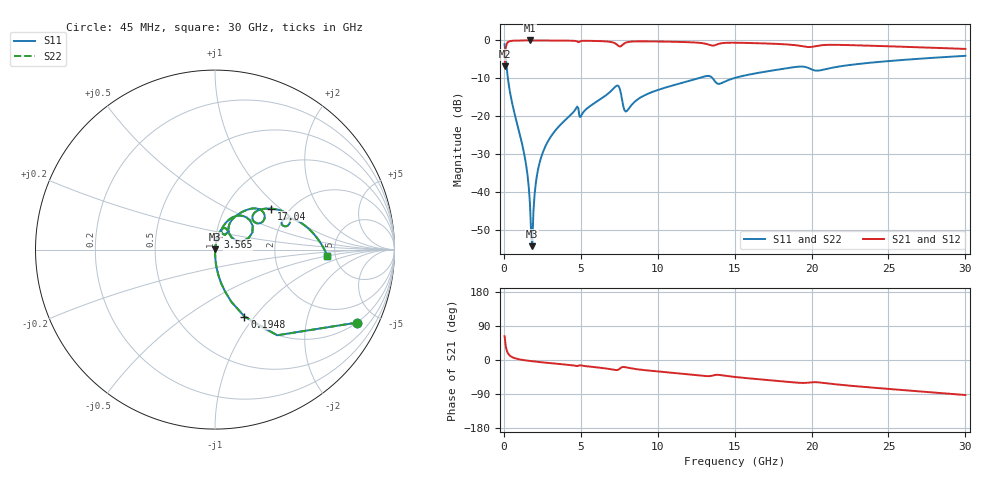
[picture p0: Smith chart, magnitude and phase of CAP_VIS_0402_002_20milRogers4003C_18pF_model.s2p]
! S-parameter model data by Modelithics Inc.  support@modelithics.com  813-866-6335  Tampa FL USA
! S-Parameter data specifications:
! Substrate: 20-mil Rogers 4003C, substrate thickness, H=0.508mm, Dielectric constant, Er=3.75
! PCB Mounting Pad Footprint: Pad width, PadW=0.50mm , Pad length, PadL=0.50mm , Pad gap, PadG (edge-to-edge)=0.40mm , Reference planes=1.4mm apart
! Created Wed Nov 18 12:52:21 2015
# hz S ma R 50
! 2 Port Network Data from SP1.SP block
! freq  magS11  angS11  magS21  angS21  magS12  angS12  magS22  angS22
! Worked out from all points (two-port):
!   401 points, 45 MHz to 30 GHz, reference 50 ohm
!   highest |S21| = -0.01 dB at 1.693 GHz (marker M1); lowest = -6.8 dB at 45 MHz (marker M2)
!   |S21| within 3 dB of the highest: 102.5 MHz to end of sweep
!   lowest |S11| = -54.3 dB at 1.842 GHz (marker M3), VSWR 1.00, Z = 50.1 + j0.128 ohm
!   |S11| at or under -10 dB: 259.5 MHz to 12.65 GHz (12.39 GHz wide, 192 % of centre); 13.56 GHz to 14.93 GHz (1.369 GHz wide, 9.61 % of centre)
!   |S22| runs from -54.3 to -1.0 dB; largest |S21 - S12| = 0
!   S11 on the Smith chart (normalised r, x): 45 MHz: 1.00, -3.90; 194.8 MHz: 1.00, -0.89; 3.565 GHz: 1.02, +0.15; 17.04 GHz: 1.63, +0.87; 30 GHz: 4.29, -0.47
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4.5e7  0.8901 -27.2  0.4556 62.8  0.4556 62.8  0.8901 -27.2
1.94775e8  0.4076 -66.2  0.9127 23.7  0.9127 23.7  0.4076 -66.2
4.194375e8  0.1947 -79.3  0.9802 10.5  0.9802 10.5  0.1947 -79.3
1.392975e9  0.02614 -88.3  0.9984 -0.9  0.9984 -0.9  0.02614 -88.3
1.54275e9  0.01602 -87.3  0.9986 -1.8  0.9986 -1.8  0.01602 -87.3
1.692525e9  0.007027 -81.9  0.9986 -2.5  0.9986 -2.5  0.007027 -81.9
1.8423e9  0.001918 41.8  0.9986 -3.3  0.9986 -3.3  0.001918 41.8
2.14185e9  0.01623 80.2  0.9983 -4.7  0.9983 -4.7  0.01623 80.2
2.366512e9  0.02626 81.0  0.998 -5.6  0.998 -5.6  0.02626 81.0
3.564712e9  0.07288 78.0  0.9952 -10.4  0.9952 -10.4  0.07288 78.0
4.688025e9  0.1264 69.5  0.9807 -15.4  0.9807 -15.4  0.1264 69.5
5.062462e9  0.1047 69.8  0.9845 -14.8  0.9845 -14.8  0.1047 69.8
7.309088e9  0.2511 45.5  0.8933 -26.5  0.8933 -26.5  0.2511 45.5
7.983075e9  0.1165 44.4  0.9438 -19.9  0.9438 -19.9  0.1165 44.4
1.007992e10  0.224 57.8  0.9673 -30.4  0.9673 -30.4  0.224 57.8
1.315031e10  0.3381 40.4  0.8998 -42.5  0.8998 -42.5  0.3381 40.4
1.397408e10  0.267 36.7  0.9009 -39.3  0.9009 -39.3  0.267 36.7
1.50225e10  0.3202 42.6  0.9321 -44.8  0.9321 -44.8  0.3202 42.6
1.704446e10  0.3883 36.0  0.9112 -52.5  0.9112 -52.5  0.3883 36.0
2.003996e10  0.4115 18.4  0.8231 -58.7  0.8231 -58.7  0.4115 18.4
2.505742e10  0.5345 12.6  0.836 -76.5  0.836 -76.5  0.5345 12.6
3e10  0.6256 -3.0  0.7719 -92.4  0.7719 -92.4  0.6256 -3.0
